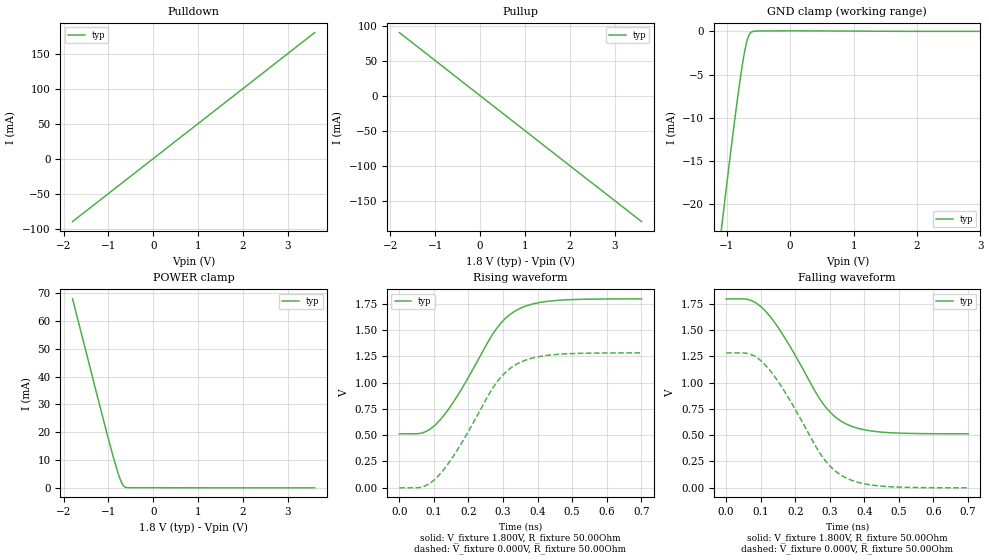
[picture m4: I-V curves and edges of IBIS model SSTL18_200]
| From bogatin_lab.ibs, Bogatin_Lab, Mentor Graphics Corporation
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[Model]   SSTL18_200
Model_type   I/O
Vinl = 650.000mV
Vinh = 1.150V
Vmeas = 900.000mV
Vref = 900.000mV
Cref = 100.000fF
Rref = 25.000Ohm
|   typ   min   max
C_comp   4.000pF   NA   NA
[Voltage Range]   1.800V   NA   NA
[Temperature Range]   50.0   NA   NA
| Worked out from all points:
|   slope of the pulldown table from 0 to 0.27 V, typ, clamps not added: 20 ohm
|   slope of the pullup table from 0 to 0.27 V, typ, clamps not added: 20 ohm
|   GND clamp passes 1 mA (typ) near -0.68 V on its own axis
|   POWER clamp passes 1 mA (typ) near -0.68 V on its own axis
|   falling waveform, V_fixture 1.800V, R_fixture 50.00Ohm: 20-80 % time 140ps typ, NA min, NA max; typ from 1.8 V to 0.512 V
|   rising waveform, V_fixture 1.800V, R_fixture 50.00Ohm: 20-80 % time 140ps typ, NA min, NA max; typ from 0.512 V to 1.8 V
|   rising waveform, V_fixture 0.000V, R_fixture 50.00Ohm: 20-80 % time 140ps typ, NA min, NA max; typ from -0.002 V to 1.28 V
|   falling waveform, V_fixture 0.000V, R_fixture 50.00Ohm: 20-80 % time 140ps typ, NA min, NA max; typ from 1.28 V to -0.002 V
[Pulldown]
|   Voltage   I(typ)   I(min)   I(max)
-1.8V     -89.85mA   NA         NA
-1.79V    -89.11mA   NA         NA
-1.76V    -87.86mA   NA         NA
3.6V      180.1mA    NA         NA
[GND Clamp]
|   Voltage   I(typ)   I(min)   I(max)
-1.8V     -68.65mA   NA         NA
-1.09V    -23.21mA   NA         NA
-1.07V    -21.97mA   NA         NA
-880mV    -10.56mA   NA         NA
-820mV    -7.212mA   NA         NA
-760mV    -4.154mA   NA         NA
-720mV    -2.411mA   NA         NA
-680mV    -1.081mA   NA         NA
-650mV    -459uA     NA         NA
-610mV    -89.94uA   NA         NA
0V        59.61uA    NA         NA
3.6V      0A         NA         NA
[Pullup]
|   Voltage   I(typ)   I(min)   I(max)
-1.8V     90.25mA    NA         NA
2.32V     -115.9mA   NA         NA
3.59V     -179mA     NA         NA
3.6V      -179.7mA   NA         NA
[POWER Clamp]
|   Voltage   I(typ)   I(min)   I(max)
-1.8V     67.89mA    NA         NA
-1.12V    24.89mA    NA         NA
-900mV    11.56mA    NA         NA
-810mV    6.555mA    NA         NA
-750mV    3.621mA    NA         NA
-700mV    1.673mA    NA         NA
-650mV    514.4uA    NA         NA
-530mV    49.71uA    NA         NA
3.6V      0A         NA         NA
[Ramp]
R_load = 50.00Ohm
|   typ   min   max
dV/dt_r   771.098mV/140.292ps   NA   NA
dV/dt_f   771.043mV/140.292ps   NA   NA
[Falling Waveform]
V_fixture = 1.800V
R_fixture = 50.00Ohm
|   Time   V(typ)   V(min)   V(max)
0s        1.797V     NA         NA
67.45ps   1.787V     NA         NA
112.4ps   1.685V     NA         NA
169.1ps   1.429V     NA         NA
276.7ps   816.7mV    NA         NA
306ps     702mV      NA         NA
339.2ps   620.3mV    NA         NA
385.2ps   561.7mV    NA         NA
446.8ps   529.5mV    NA         NA
700.9ps   512.3mV    NA         NA
[Rising Waveform]
V_fixture = 1.800V
R_fixture = 50.00Ohm
|   Time   V(typ)   V(min)   V(max)
0s        512.3mV    NA         NA
67.45ps   522.7mV    NA         NA
112.4ps   625.2mV    NA         NA
169.1ps   880.4mV    NA         NA
276.7ps   1.493V     NA         NA
306ps     1.608V     NA         NA
339.2ps   1.689V     NA         NA
385.2ps   1.748V     NA         NA
446.8ps   1.78V      NA         NA
700.9ps   1.797V     NA         NA
[Rising Waveform]
V_fixture = 0.000V
R_fixture = 50.00Ohm
|   Time   V(typ)   V(min)   V(max)
0s        -2.068mV   NA         NA
67.45ps   8.104mV    NA         NA
112.4ps   110.6mV    NA         NA
169.1ps   365.8mV    NA         NA
276.7ps   978.6mV    NA         NA
306ps     1.093V     NA         NA
339.2ps   1.175V     NA         NA
385.2ps   1.234V     NA         NA
446.8ps   1.266V     NA         NA
700.9ps   1.283V     NA         NA
[Falling Waveform]
V_fixture = 0.000V
R_fixture = 50.00Ohm
|   Time   V(typ)   V(min)   V(max)
0s        1.283V     NA         NA
67.45ps   1.273V     NA         NA
112.4ps   1.17V      NA         NA
169.1ps   915mV      NA         NA
276.7ps   302.3mV    NA         NA
306ps     187.6mV    NA         NA
339.2ps   105.9mV    NA         NA
385.2ps   47.3mV     NA         NA
446.8ps   15.17mV    NA         NA
700.9ps   -2.068mV   NA         NA
